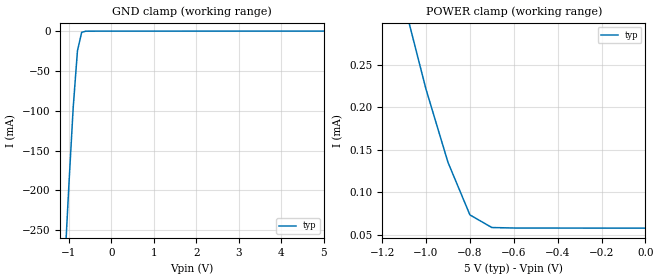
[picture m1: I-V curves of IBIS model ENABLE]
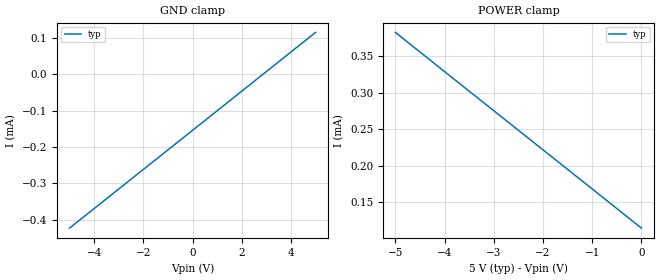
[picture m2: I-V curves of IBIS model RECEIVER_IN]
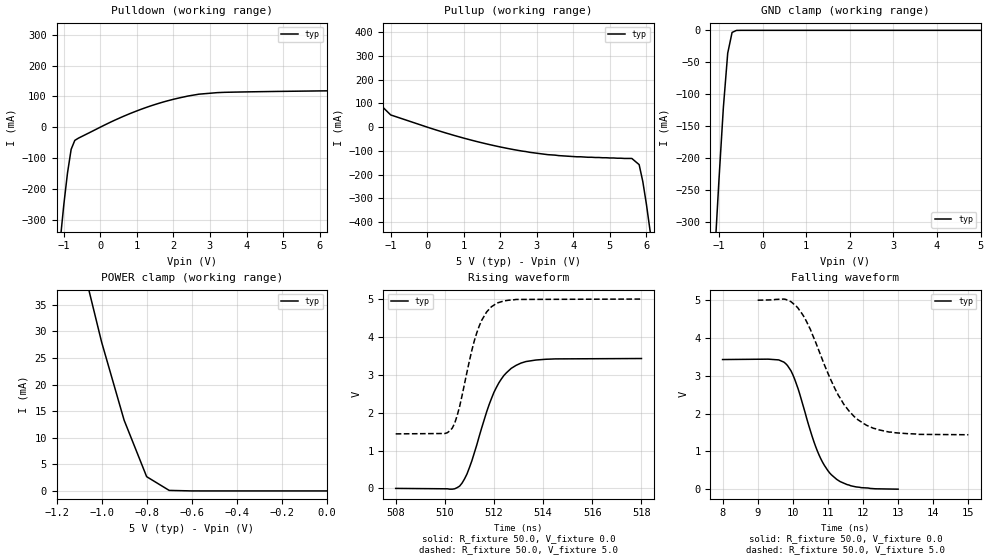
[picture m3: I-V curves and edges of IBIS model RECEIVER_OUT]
|   Texas Instruments Incorporated
|   Data Transmissions Products
|   IBIS Model for SN75LBC175A
|   16N PDIP Package
[IBIS Ver]   3.2
[Comment char]   |_char
[File name]   lbc175an.ibs
[File Rev]   2.0
[Date]   10Jan01
[Source]   File originated at Texas Instruments Incorporated.
   Data Transmission Products Group. All data based on
   Bench Measurements.
[Notes]
[Disclaimer]
(C) Copyright Texas Instruments Incorporated 2001
   All rights reserved
  Texas Instruments Incorporated hereby grants the user of this IBIS
model a non-exclusive, nontransferable license to use this IBIS model
under the following terms.  Before using this IBIS model, the user
should read this license.  If the user does not accept these terms,
the IBIS model should be returned to Texas Instruments within 30 days.
  The user is granted this license only to use the IBIS model and
is not granted rights to sell, load, rent, lease or license the IBIS
model in whole or in part, or in modified form to anyone other than
user.  User may modify the IBIS model to suit its specific applications
but rights to derivative works and such modifications shall belong to
Texas Instruments.
  This IBIS model is provided on an "AS IS" basis and Texas Instruments
makes absolutely no warranty with respect to the information contained
herein.  TEXAS INSTRUMENTS DISCLAIMS AND CUSTOMER WAIVES ALL WARRANTIES,
EXPRESS OR IMPLIED, INCLUDING WARRANTIES OF MERCHANTABILITY OR FITNESS
FOR A PARTICULAR PURPOSE. The entire risk as to quality and performance
is with the Customer. ACCORDINGLY, IN NO EVENT SHALL THE COMPANY BE LIABLE
FOR ANY DAMAGES, WHETHER IN CONTRACT OR TORT,INCLUDING ANY LOST PROFITS
OR OTHER INCIDENTAL, CONSEQUENTIAL, EXEMPLARY, OR PUNITIVE DAMAGES ARISING
OUT OF THE USE OR APPLICATION OF THE IBIS model provided in this package.
Further, Texas Instruments reserves the right to discontinue or make changes
without notice to any product herein to improve reliability, function, or
design. Texas Instruments does not convey any license under patent rights
or any other intellectual property rights, including those of third parties.
Contact Texas Instruments at ATTN:DATA TRANSMISSIONS
[Copyright]   Copyright 2001, Texas Instruments, All Rights Reserved
[Component]   SN75LBC175AN
[Manufacturer]  Texas Instruments Incorporated
[Package]
|   typ   min   max
R_pkg   0.056   0.052   0.063
L_pkg   7.637nH   5.451nH   10.525nH
C_pkg   0.528pF   0.335pF   0.893pF
[Pin]   signal_name   model_name   R_pin   L_pin   C_pin
1   1B   RECEIVER_IN   0.058   10.525n   0.892p
2   1A   RECEIVER_IN   0.062   8.759n   0.535p
3   1Y   RECEIVER_OUT   0.052   7.146n   0.387p
4   1,2EN   ENABLE   0.053   5.451n   0.408p
5   2Y   RECEIVER_OUT   0.053   5.513n   0.370p
6   2A   RECEIVER_IN   0.053   6.304n   0.336p
7   2B   RECEIVER_IN   0.057   7.830n   0.503p
8   GND   GND   0.056   9.581n   0.805p
9   3B   RECEIVER_IN   0.058   9.603n   0.807p
10   3A   RECEIVER_IN   0.062   7.864n   0.503p
11   3Y   RECEIVER_OUT   0.052   6.295n   0.335p
12   3,4EN   ENABLE   0.053   5.499n   0.356p
13   4Y   RECEIVER_OUT   0.053   5.452n   0.404p
14   4A   RECEIVER_IN   0.053   7.156n   0.387p
15   4B   RECEIVER_IN   0.063   8.740n   0.534p
16   VCC   POWER   0.056   10.478n   0.893p
[Diff_pin]   inv_pin   vdiff   tdelay_typ   tdelay_min   tdelay_max
| The 'xA' pin is Diff_pin and the 'xB' pin is the inv_pin
2   1   200mV   0 0 0   | Vth  +/-200mV
6   7   200mV   0 0 0
10   9   200mV   0 0 0
14   15   200mV   0 0 0
| Models and submodels in the file (3): ENABLE (Input), RECEIVER_IN (Input), RECEIVER_OUT (3-state)
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|   Receiver Enable Model
[Model]   ENABLE
Model_type   Input
|Signals   1,2EN,3,4EN
Vinh = 2.0
Vinl = 0.8
|   typ   min   max
C_comp   1.0pF   NA   NA
|   typ   min   max
[Temperature Range]   25.0   NA   NA
[Voltage range]   5.0V   4.75V   5.25V
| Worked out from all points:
|   GND clamp passes 1 mA (typ) near -0.67 V on its own axis
[GND_clamp]
|   Voltage   I(typ)   I(min)   I(max)
-5V       -4.21A     NA         NA
-2V       -1.22A     NA         NA
-1V       -192mA     NA         NA
-900mV    -96.1mA    NA         NA
-800mV    -24.8mA    NA         NA
-700mV    -1.47mA    NA         NA
-500mV    -17.2uA    NA         NA
5V        57.8uA     NA         NA
[Power_clamp]
| Note that the[POWER_clamp]voltage table is referenced to Vcc
| and is calculated using Vtable=Vcc - Vmeasured.
|   Voltage   I(typ)   I(min)   I(max)
-5V       4.391mA    NA         NA
-2V       1.232mA    NA         NA
-1V       221.2uA    NA         NA
-900mV    135.3uA    NA         NA
-800mV    73.39uA    NA         NA
-700mV    58.53uA    NA         NA
0V        57.8uA     NA         NA
|   Receiver Input Model
[Model]   RECEIVER_IN
Model_type   Input
|Signals   1A,1B,2A,2B,3A,3B,4A,4B
Vinh = 2.0
Vinl = 0.8
|   typ   min   max
C_comp   1.0pF   NA   NA
|   typ   min   max
[Temperature Range]   25.0   NA   NA
[Voltage range]   5.0V   4.75V   5.25V
[GND_clamp]
|   Voltage   I(typ)   I(min)   I(max)
-5V       -422.5uA   NA         NA
0V        -154.3uA   NA         NA
5V        114.3uA    NA         NA
[Power_clamp]
| Note that the[POWER_clamp]voltage table is referenced to Vcc
| and is calculated using Vtable=Vcc - Vmeasured.
|   Voltage   I(typ)   I(min)   I(max)
-5V       382.5uA    NA         NA
-4V       328.8uA    NA         NA
-3V       275.2uA    NA         NA
-2V       221.6uA    NA         NA
-1V       168uA      NA         NA
0V        114.3uA    NA         NA
|   Receiver Output Model
[Model]   RECEIVER_OUT
Model_type   3-state
| Signals   1Y,2Y,3Y,4Y
Vmeas = 1.5V   |Reference voltage for timing measurements
Cref = 15pF   |Timing specification test load capacitance value
Vref = 0   |Timing specification test load voltage; GND
| variable   typ   min   max
C_comp   1.0pF   NA   NA
|   typ   min   max
[Temperature Range]   25.0   NA   NA
[Voltage range]   5.0V   4.75V   5.25V
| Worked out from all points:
|   slope of the pulldown table from 0 to 0.75 V, typ, clamps not added: 18.3 ohm
|   slope of the pullup table from 0 to 0.75 V, typ, clamps not added: 21.1 ohm
|   GND clamp passes 1 mA (typ) near -0.63 V on its own axis
|   POWER clamp passes 1 mA (typ) near -0.73 V on its own axis
|   rising waveform, R_fixture 50.0, V_fixture 0.0: 20-80 % time 1.09ns typ, NA min, NA max; typ from 0 V to 3.43 V
|   falling waveform, R_fixture 50.0, V_fixture 0.0: 20-80 % time 747ps typ, NA min, NA max; typ from 3.43 V to 0 V
|   rising waveform, R_fixture 50.0, V_fixture 5.0: 20-80 % time 802ps typ, NA min, NA max; typ from 1.44 V to 5 V
|   falling waveform, R_fixture 50.0, V_fixture 5.0: 20-80 % time 1.06ns typ, NA min, NA max; typ from 5 V to 1.44 V
[Pulldown]
|   Voltage   I(typ)   I(min)   I(max)
-5V       -4.96A     NA         NA
-2V       -1.44A     NA         NA
-1V       -251mA     NA         NA
-900mV    -149mA     NA         NA
-800mV    -72.1mA    NA         NA
-700mV    -43mA      NA         NA
400mV     22.9mA     NA         NA
2.7V      107mA      NA         NA
6.3V      118mA      NA         NA
6.6V      139mA      NA         NA
7.7V      328mA      NA         NA
10V       741mA      NA         NA
[Pullup]
|   Voltage   I(typ)   I(min)   I(max)
| Note that the[Pullup]voltage table is referenced to Vcc
| and is calculated using Vtable=Vcc - Vmeasured.
-5V       740mA      NA         NA
-4V       560mA      NA         NA
-3V       380mA      NA         NA
-2V       202mA      NA         NA
-1V       51.4mA     NA         NA
2.4V      -95.6mA    NA         NA
5.6V      -132mA     NA         NA
5.8V      -158mA     NA         NA
5.9V      -229mA     NA         NA
6V        -326mA     NA         NA
7V        -1.44A     NA         NA
10V       -4.96A     NA         NA
| Output in High Impedance (off)
[GND_clamp]
|   Voltage   I(typ)   I(min)   I(max)
-5V       -4.96A     NA         NA
-2V       -1.44A     NA         NA
-1V       -233mA     NA         NA
-900mV    -121mA     NA         NA
-800mV    -35.7mA    NA         NA
-700mV    -3.28mA    NA         NA
-600mV    -151uA     NA         NA
5V        66.5pA     NA         NA
[POWER_clamp]
|   Voltage   I(typ)   I(min)   I(max)
| Note that the [POWER_clamp] voltage table is referenced to Vcc
| and is calculated using Vtable = Vcc - Vmeasured.
| Outputs in Tri-state.
-5V       740mA      NA         NA
-2V       201mA      NA         NA
-1V       28mA       NA         NA
-900mV    13.3mA     NA         NA
-800mV    2.68mA     NA         NA
-700mV    98.5uA     NA         NA
0V        66.5pA     NA         NA
[Ramp]
|   typ   min   max
dV/dt_r   2.54v/1.2ns   NA   NA
dV/dt_f   2.14v/1.0ns   NA   NA
R_load = 50Ohm
[Rising Waveform]
R_fixture = 50.0
V_fixture = 0.0
C_fixture = 0p
L_fixture = 0n
|   V(typ)   V(min)   V(max)
508ns     0V         NA         NA
510.3ns   -20mV      NA         NA
510.6ns   60mV       NA         NA
511ns     550mV      NA         NA
511.7ns   2.02V      NA         NA
512ns     2.54V      NA         NA
512.4ns   2.98V      NA         NA
512.9ns   3.25V      NA         NA
514.1ns   3.41V      NA         NA
518ns     3.43V      NA         NA
[Falling Waveform]
R_fixture = 50.0
V_fixture = 0.0
C_fixture = 0p
L_fixture = 0n
|   V(typ)   V(min)   V(max)
8ns       3.43V      NA         NA
9.3ns     3.44V      NA         NA
9.75ns    3.36V      NA         NA
9.95ns    3.13V      NA         NA
10.05ns   2.92V      NA         NA
10.65ns   1.13V      NA         NA
10.85ns   710mV      NA         NA
11.05ns   430mV      NA         NA
11.65ns   90mV       NA         NA
13ns      0V         NA         NA
[Rising Waveform]
R_fixture = 50.0
V_fixture = 5.0
C_fixture = 0p
L_fixture = 0n
|   V(typ)   V(min)   V(max)
508ns     1.44V      NA         NA
510ns     1.45V      NA         NA
510.3ns   1.59V      NA         NA
510.6ns   2.16V      NA         NA
511.1ns   3.65V      NA         NA
511.3ns   4.11V      NA         NA
511.7ns   4.66V      NA         NA
512.1ns   4.89V      NA         NA
512.9ns   4.99V      NA         NA
518ns     5V         NA         NA
[Falling Waveform]
R_fixture = 50.0
V_fixture = 5.0
C_fixture = 0p
L_fixture = 0n
|   V(typ)   V(min)   V(max)
9ns       5V         NA         NA
9.75ns    5.03V      NA         NA
10.15ns   4.79V      NA         NA
10.5ns    4.23V      NA         NA
11.05ns   2.96V      NA         NA
11.3ns    2.48V      NA         NA
11.6ns    2.07V      NA         NA
12ns      1.74V      NA         NA
12.75ns   1.51V      NA         NA
15ns      1.44V      NA         NA
